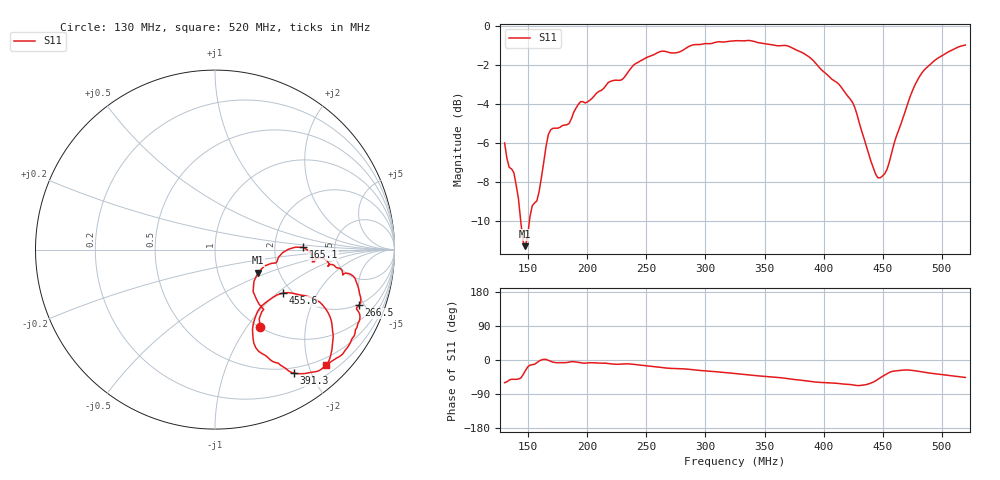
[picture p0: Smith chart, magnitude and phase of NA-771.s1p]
!Agilent N9912A: A.05.34
!Date: Friday, 14 June 2013 16:44:21
!Model: N9912A
!Serial: MY50492702
!CABLE_LOSS: 0.000
!CABLE_NAME:
!VELOCITY_FACTOR: 1.000000000
!GPS Latitude:
!GPS Longitude:
!GPS TimeStamp: 0001-01-01 00:00:00Z
!GPS Seconds Since Last Read: 0
!CHECKSUM:1933835031
!Correction: S11(ON*)
!S1P File: Measurement: S11:
# Hz S DB R 50
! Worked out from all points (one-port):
!   201 points, 130 MHz to 520 MHz, reference 50 ohm
!   lowest |S11| = -11.3 dB at 147.6 MHz (marker M1), VSWR 1.75, Z = 77.8 - j21.7 ohm
!   |S11| at or under -10 dB: 143.6 MHz to 151 MHz (7.414 MHz wide, 5.03 % of centre)
!   S11 on the Smith chart (normalised r, x): 130 MHz: 1.00, -1.16; 165.1 MHz: 2.93, +0.10; 266.5 MHz: 1.92, -4.59; 391.3 MHz: 0.42, -1.74; 455.6 MHz: 1.79, -1.08; 520 MHz: 0.36, -2.30
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1.3e8  -6.00 -59.8
1.339e8  -7.26 -53.1
1.417e8  -8.86 -50.2
1.456e8  -11.06 -39.1
1.4755e8  -11.31 -28.3
1.534e8  -9.23 -12.5
1.5925e8  -8.49 -2.7
1.651e8  -6.17 1.4
1.7095e8  -5.25 -5.7
1.7875e8  -5.11 -7.0
1.885e8  -4.42 -4.4
1.963e8  -3.88 -8.2
2.275e8  -2.79 -11.1
2.4115e8  -1.91 -12.2
2.665e8  -1.30 -21.1
2.7625e8  -1.36 -22.8
2.899e8  -0.96 -25.8
3.25e8  -0.75 -35.7
3.7375e8  -1.13 -50.9
3.913e8  -1.77 -57.5
4.225e8  -3.75 -64.7
4.303e8  -4.99 -67.5
4.381e8  -6.57 -63.1
4.459e8  -7.79 -51.0
4.5565e8  -6.97 -32.8
4.7125e8  -3.97 -26.3
4.849e8  -2.27 -32.3
5.2e8  -0.97 -46.1
